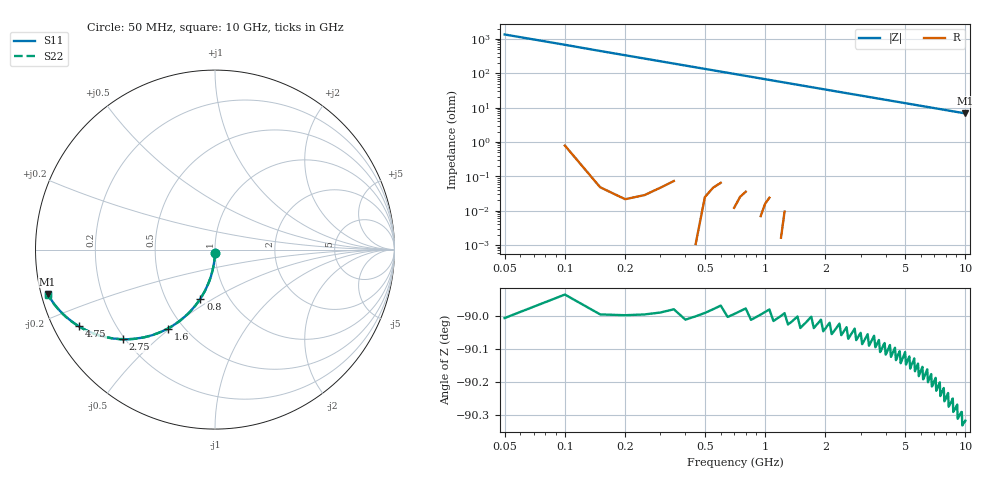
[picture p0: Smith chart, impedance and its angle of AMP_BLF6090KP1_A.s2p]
! Created Tue Sep  1 15:40:54 2009
# ghz S ma R 50
! 2 Port Network Data from SP1.SP block
! freq  magS11  angS11  magS21  angS21  magS12  angS12  magS22  angS22
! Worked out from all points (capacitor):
!   200 points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, 50 MHz to 10 GHz, reference 50 ohm
!   read as one part in shunt: C = 2.38 pF near 100 MHz
!   lowest |Z| = 6.76 ohm at 10 GHz (marker M1)
!   S11 on the Smith chart (normalised r, x): 50 MHz: 1.00, -0.04; 800 MHz: 0.74, -0.44; 1.6 GHz: 0.41, -0.49; 2.75 GHz: 0.19, -0.39; 4.75 GHz: 0.07, -0.26; 10 GHz: 0.02, -0.13
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0.05  0.01834 -91.0  0.9998 -1.1  0.9998 -1.1  0.01864 -91.0
0.1  0.03663 -92.2  0.9992 -2.1  0.9992 -2.1  0.03721 -92.1
0.15  0.05648 -93.2  0.9984 -3.2  0.9984 -3.2  0.05591 -93.2
0.2  0.07463 -94.2  0.9972 -4.3  0.9972 -4.3  0.07434 -94.3
0.25  0.09269 -95.3  0.9956 -5.3  0.9956 -5.3  0.09267 -95.3
0.35  0.1288 -97.5  0.9915 -7.5  0.9915 -7.5  0.1294 -97.4
0.45  0.1656 -99.5  0.9861 -9.5  0.9861 -9.5  0.1654 -99.5
0.65  0.2358 -103.6  0.9717 -13.6  0.9717 -13.6  0.2354 -103.6
0.8  0.2852 -106.7  0.9581 -16.6  0.9581 -16.6  0.2857 -106.6
0.95  0.3336 -109.5  0.9425 -19.5  0.9425 -19.5  0.3336 -109.5
1.15  0.3939 -113.2  0.919 -23.2  0.919 -23.2  0.3938 -113.2
1.6  0.512 -120.8  0.8588 -30.9  0.8588 -30.9  0.512 -120.8
1.75  0.5465 -123.1  0.8375 -33.2  0.8375 -33.2  0.5461 -123.1
2.15  0.6256 -128.7  0.7804 -38.8  0.7804 -38.8  0.625 -128.7
2.75  0.7152 -135.8  0.6985 -45.8  0.6985 -45.8  0.7155 -135.7
3.4  0.7846 -141.8  0.6199 -51.8  0.6199 -51.8  0.7847 -141.7
4.05  0.8335 -146.5  0.5529 -56.6  0.5529 -56.6  0.8333 -146.5
4.75  0.8706 -150.6  0.4926 -60.7  0.4926 -60.7  0.8703 -150.5
5.05  0.8829 -152.1  0.4701 -62.2  0.4701 -62.2  0.8828 -152.0
6.7  0.9276 -158.3  0.3731 -68.4  0.3731 -68.4  0.928 -158.1
8.35  0.9515 -162.3  0.3076 -72.5  0.3076 -72.5  0.9517 -162.1
10  0.965 -165.2  0.2611 -75.4  0.2611 -75.4  0.9655 -164.9
